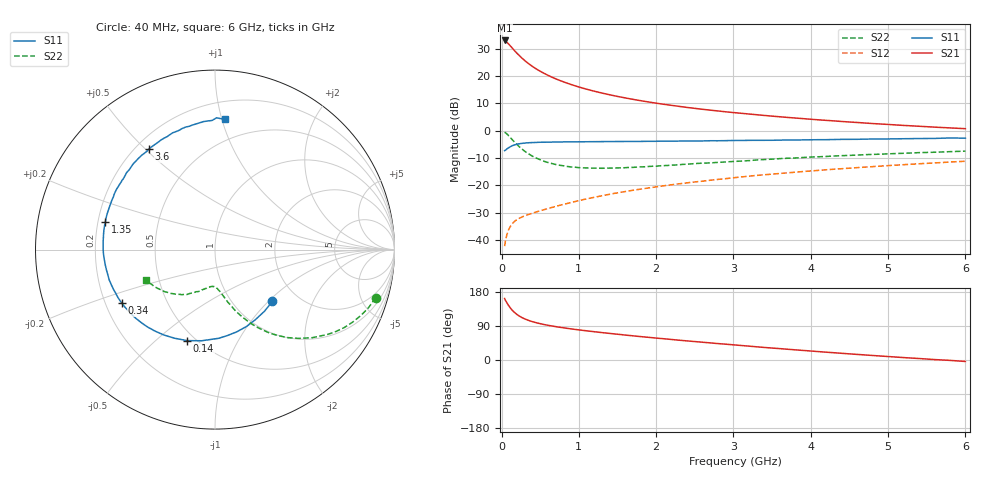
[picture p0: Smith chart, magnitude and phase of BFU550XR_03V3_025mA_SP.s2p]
! Filename:  P:\Prog\Test\Noise\ATS_data\Testdata_Net\03 Spar\BFU550XR_APG2013_45_C05_03p3V_025mA_SP_CM01_D.s2p
! Date/Time: Tue 06/Aug/2013 14:38:15
! BFU550XR_APG2013_45_C05_03p3V_25to35mA_SP_CM01_Bias1_R.s2p
! MDIF S-parameter v. bias file
! BFU550XR_APG2013_45_C05_03p3V_25to35mA_SP_CM01
! Date/time Mon Aug 05 16:35:29 2013
! bias mode 1
! bias variable = I_out
! VAR bias_var= 1
! VAR V_out= 3.3000
! VAR I_out= 25.0050
! VAR V_in= 0.8463
! VAR I_in= 0.2886
! Device data file deembeded for feedlines and parallel
! Original file: \03 Spar\BFU550XR_APG2013_45_C05_03p3V_025mA_SP_CM01_R.s2p
! Feed-files: PR006V01_02082013_Feed1.s2p, PR006V01_02082013_Feed2.s2p
! Parallel-file: PR006V01_02082013_Par.s2p
# MHz S MA R 50
!  Freq-MHz  S11-mag  S11-arg  S21-mag  S21-arg  S12-mag  S12-arg  S22-mag  S22-arg
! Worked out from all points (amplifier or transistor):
!   98 points, 40 MHz to 6 GHz, reference 50 ohm
!   highest |S21| = 33.0 dB at 40 MHz (marker M1)
!   |S21| within 3 dB of that: start of sweep to 146 MHz
!   unconditionally stable (mu >= 1): 1.223 GHz to 3.06 GHz
!   at 300 MHz: K = 0.52, MSG = 28.4 dB, |S12| = -31.1 dB
!   at 1.6 GHz: K = 1.03, MAG = 16.0 dB, |S12| = -22.3 dB
!   at 6 GHz: K = 0.85, MSG = 6.0 dB, |S12| = -11.2 dB
!   S11 on the Smith chart (normalised r, x): 40 MHz: 1.49, -1.06; 140 MHz: 0.45, -0.64; 340 MHz: 0.27, -0.25; 1.35 GHz: 0.23, +0.12; 3.6 GHz: 0.25, +0.51; 6 GHz: 0.33, +1.02
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40  0.4309 -42.1  44.44 162.3  0.007734 76.2  0.9342 -16.6
50  0.4402 -51.1  43.19 157.7  0.00946 73.6  0.9151 -20.6
80  0.4739 -75.1  39.79 147.4  0.01396 66.1  0.8411 -31.1
100  0.4946 -87.6  37.17 141.3  0.01634 61.9  0.7848 -37.0
120  0.5134 -98.3  34.62 135.8  0.01831 58.6  0.7311 -42.2
140  0.5303 -107.0  32.18 131.1  0.01997 56.0  0.6807 -46.6
160  0.5429 -114.6  29.82 127.0  0.0214 53.8  0.6359 -50.5
180  0.5545 -120.9  27.79 123.3  0.02262 52.1  0.5934 -53.8
220  0.5722 -131.1  24.31 117.2  0.0246 50.0  0.5227 -59.2
280  0.5887 -142.2  20.21 110.4  0.02697 48.7  0.4425 -65.2
340  0.5986 -150.1  17.19 105.3  0.02907 48.7  0.3852 -69.4
460  0.6097 -161.0  13.14 97.9  0.03299 50.1  0.3103 -75.4
650  0.6172 -172.1  9.511 89.8  0.03936 53.6  0.2507 -81.2
850  0.6229 -179.9  7.356 83.5  0.04666 56.4  0.2215 -86.0
1050  0.6254 173.9  5.985 78.2  0.05451 58.5  0.2091 -89.2
1350  0.6303 166.1  4.679 71.2  0.06666 60.0  0.2062 -94.3
2050  0.6409 151.2  3.098 57.0  0.09579 59.9  0.2278 -104.9
3100  0.6616 131.6  2.074 38.3  0.1424 55.6  0.2774 -118.8
3600  0.6706 123.2  1.79 30.0  0.1648 52.3  0.3077 -125.6
4100  0.6827 114.6  1.575 22.1  0.1877 48.7  0.3326 -131.7
5200  0.711 97.2  1.245 6.4  0.2384 40.0  0.3854 -145.9
6000  0.7274 85.8  1.086 -3.9  0.2754 32.8  0.4218 -156.5
